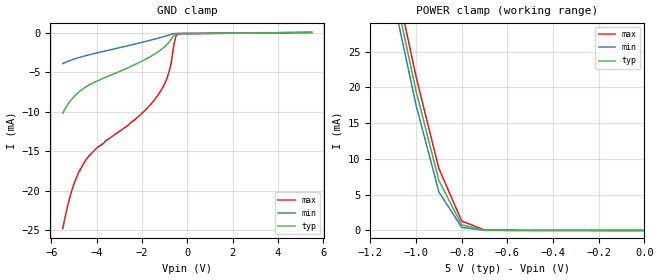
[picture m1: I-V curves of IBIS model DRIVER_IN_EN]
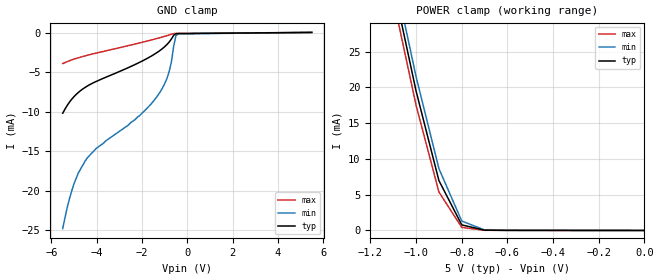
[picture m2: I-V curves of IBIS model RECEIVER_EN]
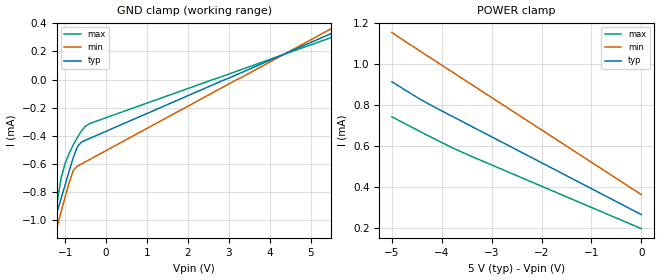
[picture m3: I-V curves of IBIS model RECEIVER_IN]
|   Texas Instruments Incorporated
|   Data Transmissions Products
|   IBIS Model for TB5T1
|   16DW SOIC Package
[IBIS Ver]   3.2
[Comment char]   |_char
[File name]   tb5t1dw.ibs
[File Rev]   1.0
[Date]   29Jan04
[Source]   File originated at Texas Instruments Incorporated.
   Data Transmission Products Group. All data based on
   Simulation.
[Notes]
[Disclaimer]
(C) Copyright Texas Instruments Incorporated 2004
   All rights reserved
  Texas Instruments Incorporated hereby grants the user of this IBIS
model a non-exclusive, nontransferable license to use this IBIS model
under the following terms.  Before using this IBIS model, the user
should read this license.  If the user does not accept these terms,
the IBIS model should be returned to Texas Instruments within 30 days.
  The user is granted this license only to use the IBIS model and
is not granted rights to sell, load, rent, lease or license the IBIS
model in whole or in part, or in modified form to anyone other than
user.  User may modify the IBIS model to suit its specific applications
but rights to derivative works and such modifications shall belong to
Texas Instruments.
  This IBIS model is provided on an "AS IS" basis and Texas Instruments
makes absolutely no warranty with respect to the information contained
herein.  TEXAS INSTRUMENTS DISCLAIMS AND CUSTOMER WAIVES ALL WARRANTIES,
EXPRESS OR IMPLIED, INCLUDING WARRANTIES OF MERCHANTABILITY OR FITNESS
FOR A PARTICULAR PURPOSE. The entire risk as to quality and performance
is with the Customer. ACCORDINGLY, IN NO EVENT SHALL THE COMPANY BE LIABLE
FOR ANY DAMAGES, WHETHER IN CONTRACT OR TORT,INCLUDING ANY LOST PROFITS
OR OTHER INCIDENTAL, CONSEQUENTIAL, EXEMPLARY, OR PUNITIVE DAMAGES ARISING
OUT OF THE USE OR APPLICATION OF THE IBIS model provided in this package.
Further, Texas Instruments reserves the right to discontinue or make changes
without notice to any product herein to improve reliability, function, or
design. Texas Instruments does not convey any license under patent rights
or any other intellectual property rights, including those of third parties.
Contact Texas Instruments at ATTN:DATA TRANSMISSIONS
[Copyright]   Copyright 2004, Texas Instruments, All Rights Reserved
[Component]   TB5T1
[Manufacturer]  Texas Instruments
[Package]
|   typ   min   max
R_pkg   0.046   0.034   0.057
L_pkg   4.858nH   3.987nH   6.214nH
C_pkg   0.715pF   0.502pF   1.046pF
[Pin]   signal_name   model_name   R_pin   L_pin   C_pin
1   RO1   RECEIVER_OUT   0.057   6.214nH   1.026pF
2   DI1   DRIVER_IN_EN   0.055   5.236nH   0.818pF
3   VCC   POWER   0.034   3.987nH   0.723pF
4   ED   DRIVER_IN_EN   0.036   3.996nH   0.726pF
5   ER   RECEIVER_EN   0.036   3.996nH   0.726pF
6   GND   GND   0.034   3.987nH   0.704pF
7   DI2   DRIVER_IN_EN   0.055   5.236nH   0.818pF
8   RO2   RECEIVER_OUT   0.057   6.214nH   1.046pF
9   RI2   RECEIVER_IN   0.057   6.214nH   0.827pF
10   RI2(-)   RECEIVER_IN   0.055   5.236nH   0.597pF
11   DO2   DRIVER_OUT   0.034   3.987nH   0.502pF
12   DO2(-)   DRIVER_OUT   0.036   3.996nH   0.505pF
13   DO1(-)   DRIVER_OUT   0.036   3.996nH   0.505pF
14   DO1   DRIVER_OUT   0.034   3.987nH   0.502pF
15   RI1(-)   RECEIVER_IN   0.055   5.236nH   0.597pF
16   RI1   RECEIVER_IN   0.057   6.214nH   0.827pF
[Diff_pin]   inv_pin   vdiff   tdelay_typ   tdelay_min   tdelay_max
| The 'RIx' or 'DOx' are diff pins and the RIx'(-) or 'DOx'(-) are inv_pins
   16   15   100mV   0   0   0
   9   10   100mV   0   0   0
   14   13   NA   0   0   0
   11   12   NA   0   0   0
| Models and submodels in the file (5): DRIVER_IN_EN (Input), RECEIVER_EN (Input), RECEIVER_IN (Input), RECEIVER_OUT (3-state), DRIVER_OUT (Output_ECL)
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|   Driver Input/Enable Model
[Model]   DRIVER_IN_EN
Model_type   Input
|Signals   DI1,DI2,ED
Vinh = 2.4
Vinl = 0.4
|   typ   min   max
C_comp   964fF   924fF   1010fF
|   typ   min   max
[Temperature Range]   25.0   -40.0   125.0
[Voltage range]   5.0V   4.5V   5.5V
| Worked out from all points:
|   GND clamp passes 1 mA (typ) near -0.75 V on its own axis
|   POWER clamp passes 1 mA (typ) near -0.80 V on its own axis
[GND_clamp]
| Voltage   I(typ)   I(min)   I(max)
-5.5V     -10.2mA    -3.93mA    -24.8mA
-5.3V     -9.21mA    -3.68mA    -22.1mA
-5V       -8.1mA     -3.36mA    -19.1mA
-4.5V     -6.92mA    -2.94mA    -16.2mA
-4V       -6.16mA    -2.59mA    -14.6mA
-2.1V     -3.76mA    -1.31mA    -10.5mA
-1.5V     -2.83mA    -876uA     -8.7mA
-1.1V     -2.04mA    -566uA     -7.04mA
-800mV    -1.21mA    -311uA     -4.96mA
-700mV    -818uA     -220uA     -3.71mA
-500mV    -158uA     -114uA     -389uA
5.5V      13.6uA     12uA       16.5uA
[Power_clamp]
| Note that the[POWER_clamp]voltage table is referenced to Vcc
| and is calculated using Vtable=Vcc - Vmeasured.
|   Voltage   I(typ)   I(min)   I(max)
-5V       324mA      323mA      330mA
-1.1V     34.4mA     32.4mA     36.4mA
-1V       19.5mA     17.5mA     21.5mA
-900mV    6.98mA     5.38mA     8.65mA
-800mV    782uA      431uA      1.32mA
-700mV    41.2uA     26.6uA     71.3uA
0V        1.02uA     1.75uA     633nA
|   Receiver Enable Model
[Model]   RECEIVER_EN
Model_type   Input
|Signals   ER
Vinh = 2.4
Vinl = 0.4
|   typ   min   max
C_comp   964fF   924fF   1010fF
|   typ   min   max
[Temperature Range]   25.0   -40   125
[Voltage range]   5.0V   4.5V   5.5V
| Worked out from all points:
|   GND clamp passes 1 mA (typ) near -0.75 V on its own axis
|   POWER clamp passes 1 mA (typ) near -0.80 V on its own axis
[GND_clamp]
| Voltage   I(typ)   I(min)   I(max)
-5.5V     -10.2mA    -24.8mA    -3.93mA
-5.3V     -9.21mA    -22.1mA    -3.68mA
-5V       -8.1mA     -19.1mA    -3.36mA
-4.5V     -6.92mA    -16.2mA    -2.94mA
-4V       -6.16mA    -14.6mA    -2.59mA
-2.1V     -3.76mA    -10.5mA    -1.31mA
-1.5V     -2.83mA    -8.7mA     -876uA
-1.1V     -2.04mA    -7.04mA    -566uA
-800mV    -1.21mA    -4.96mA    -311uA
-700mV    -818uA     -3.71mA    -220uA
-500mV    -158uA     -389uA     -114uA
5.5V      13.6uA     16.5uA     12uA
[Power_clamp]
| Note that the[POWER_clamp]voltage table is referenced to Vcc
| and is calculated using Vtable=Vcc - Vmeasured.
|   Voltage   I(typ)   I(min)   I(max)
-5V       324mA      330mA      323mA
-1.1V     34.4mA     36.4mA     32.4mA
-1V       19.5mA     21.5mA     17.5mA
-900mV    6.98mA     8.65mA     5.38mA
-800mV    782uA      1.32mA     431uA
-700mV    41.2uA     71.3uA     26.6uA
0V        1.02uA     633nA      1.75uA
|   Receiver Input Model
[Model]   RECEIVER_IN
Model_type   Input
|Signals   RI1,RI1(-),RI2,RI2(-)
Vinh = 3.3
Vinl = 3.1
|   typ   min   max
C_comp   61.4fF   61.4fF   61.4fF
|   typ   min   max
[Temperature Range]   25.0   -40   125
[Voltage range]   5.0V   4.5V   5.5V
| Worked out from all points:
|   GND clamp passes 1 mA (typ) near -1.25 V on its own axis
[GND_clamp]
| Voltage   I(typ)   I(min)   I(max)
-5.5V     -73.88mA   -133.6mA   -75.47mA
-1.4V     -1.14mA    -1.266mA   -1.771mA
-1.3V     -1.044mA   -1.158mA   -1.213mA
-1.2V     -946.3uA   -1.05mA    -884.2uA
-1.1V     -847.6uA   -941.8uA   -702.9uA
-1V       -748.1uA   -834.3uA   -596.2uA
-900mV    -648.8uA   -730.7uA   -522.6uA
-800mV    -553.4uA   -645.9uA   -463.3uA
-700mV    -475.5uA   -614.8uA   -411uA
-600mV    -443.7uA   -598.8uA   -364.9uA
-500mV    -430.2uA   -583uA     -330.1uA
5.5V      327.2uA    361.6uA    298.8uA
[Power_clamp]
| Note that the[POWER_clamp]voltage table is referenced to Vcc
| and is calculated using Vtable=Vcc - Vmeasured.
|   Voltage   I(typ)   I(min)   I(max)
-5V       912.2uA    1.153mA    740.9uA
-4.4V     822.4uA    1.056mA    665uA
-3.6V     719.4uA    929.9uA    569uA
0V        263.9uA    361.6uA    195.2uA
